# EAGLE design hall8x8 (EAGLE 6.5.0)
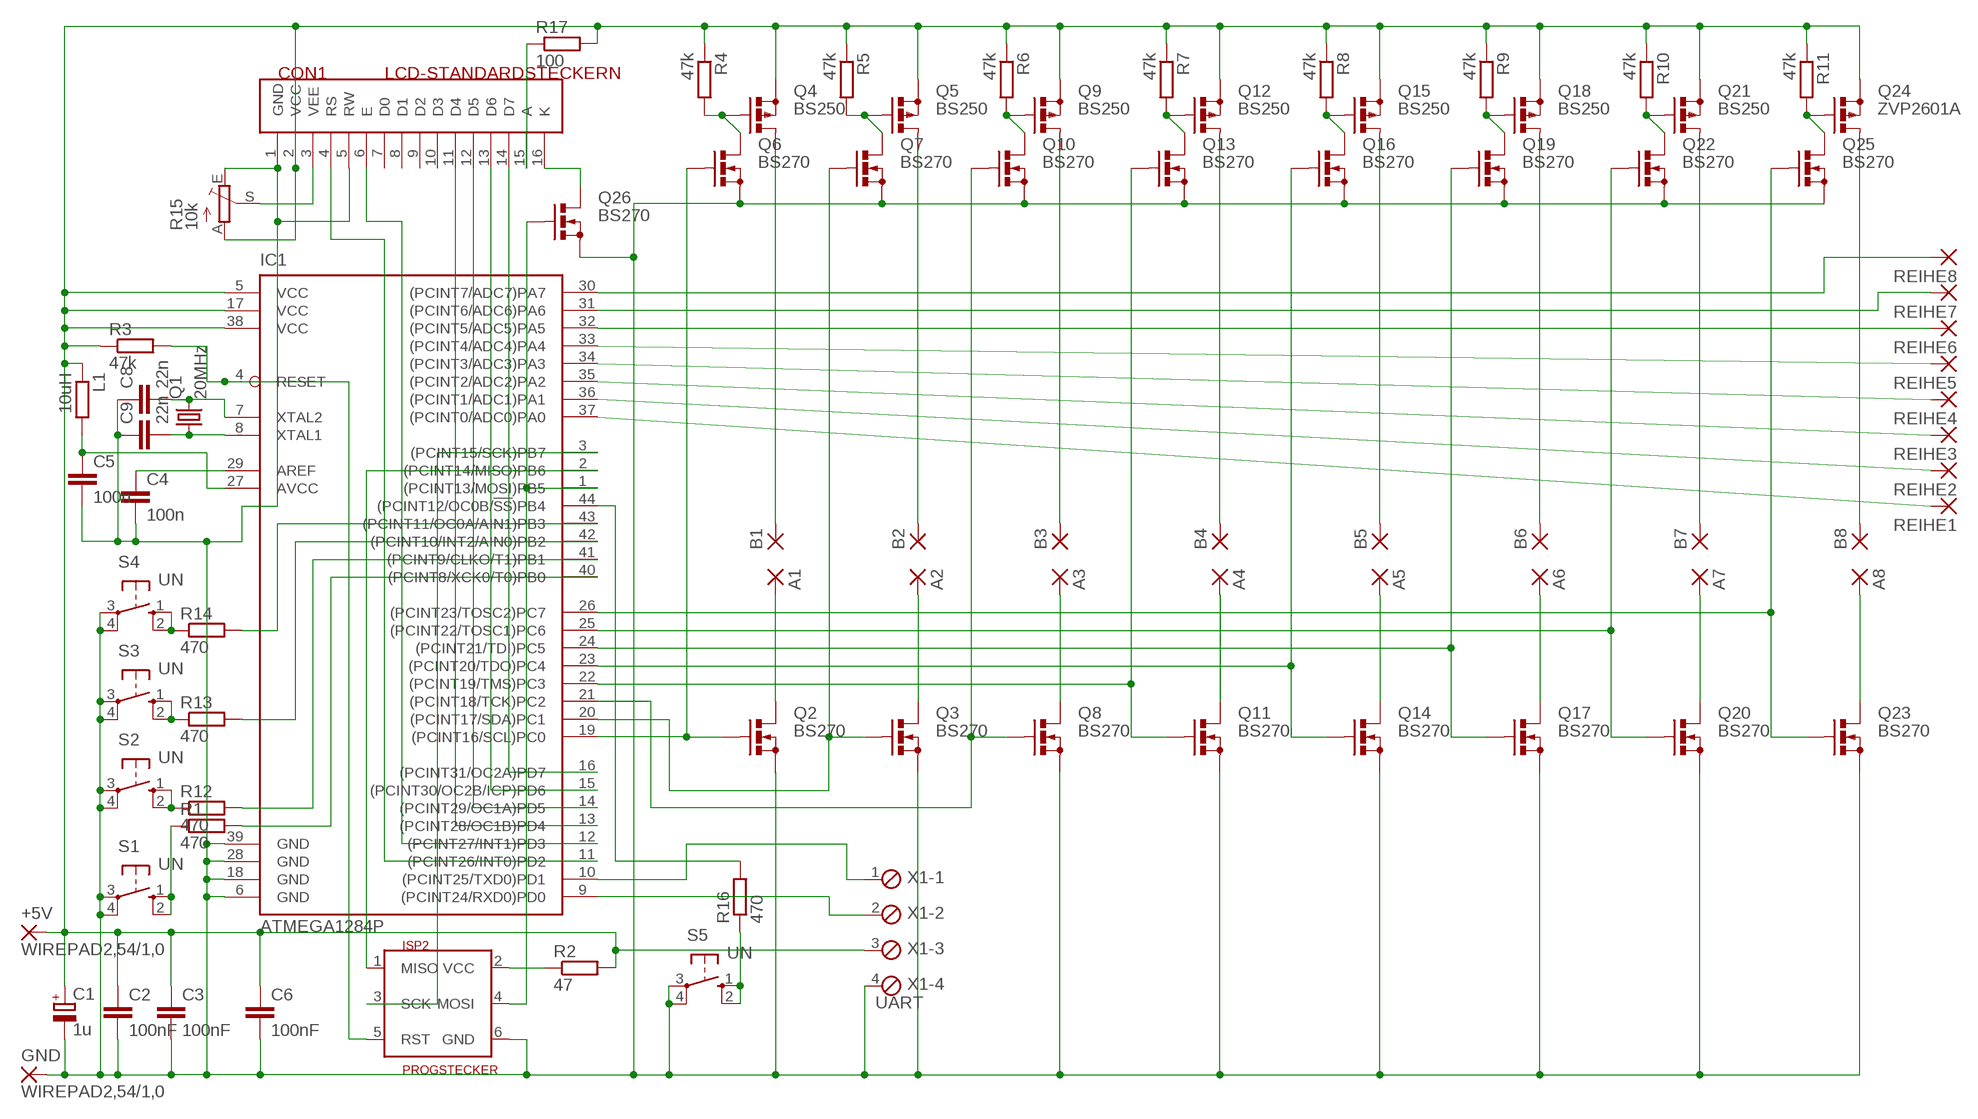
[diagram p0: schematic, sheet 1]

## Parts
+5V  WIREPAD2,54/1,0  [2,54/1,0]
A1  WIREPAD2,15/1,0  [2,15/1,0]
A2  WIREPAD2,15/1,0  [2,15/1,0]
A3  WIREPAD2,15/1,0  [2,15/1,0]
A4  WIREPAD2,15/1,0  [2,15/1,0]
A5  WIREPAD2,15/1,0  [2,15/1,0]
A6  WIREPAD2,15/1,0  [2,15/1,0]
A7  WIREPAD2,15/1,0  [2,15/1,0]
A8  WIREPAD2,15/1,0  [2,15/1,0]
B1  WIREPAD2,15/1,0  [2,15/1,0]
B2  WIREPAD2,15/1,0  [2,15/1,0]
B3  WIREPAD2,15/1,0  [2,15/1,0]
B4  WIREPAD2,15/1,0  [2,15/1,0]
B5  WIREPAD2,15/1,0  [2,15/1,0]
B6  WIREPAD2,15/1,0  [2,15/1,0]
B7  WIREPAD2,15/1,0  [2,15/1,0]
B8  WIREPAD2,15/1,0  [2,15/1,0]
C1  1u  CPOL-EUE5-6  [E5-6]
C2  100nF  C-EU025-025X050  [C025-025X050]
C3  100nF  C-EU025-025X050  [C025-025X050]
C4  100n  C-EUC1206  [C1206]
C5  100n  C-EUC1206  [C1206]
C6  100nF  C-EU025-025X050  [C025-025X050]
C8  22n  C-EUC1206  [C1206]
C9  22n  C-EUC1206  [C1206]
CON1  LCD-STANDARDSTECKERN  [STECKER16]
GND  WIREPAD2,54/1,0  [2,54/1,0]
IC1  ATMEGA1284P  ATMEGA644A  [TQFP44]
ISP2  PROGSTECKER  ISP6N  [ISP6]
L1  10uH  R-EU_0204/7  [0204/7]
Q1  20MHz  CRYSTALHC49S  [HC49/S]
Q2  BS270  BS170  [SOT54E]
Q3  BS270  BS170  [SOT54E]
Q4  BS250  [SOT54E]
Q5  BS250  [SOT54E]
Q6  BS270  BS170  [SOT54E]
Q7  BS270  BS170  [SOT54E]
Q8  BS270  BS170  [SOT54E]
Q9  BS250  [SOT54E]
Q10  BS270  BS170  [SOT54E]
Q11  BS270  BS170  [SOT54E]
Q12  BS250  [SOT54E]
Q13  BS270  BS170  [SOT54E]
Q14  BS270  BS170  [SOT54E]
Q15  BS250  [SOT54E]
Q16  BS270  BS170  [SOT54E]
Q17  BS270  BS170  [SOT54E]
Q18  BS250  [SOT54E]
Q19  BS270  BS170  [SOT54E]
Q20  BS270  BS170  [SOT54E]
Q21  BS250  [SOT54E]
Q22  BS270  BS170  [SOT54E]
Q23  BS270  BS170  [SOT54E]
Q24  ZVP2601A  BS250  [SOT54E]
Q25  BS270  BS170  [SOT54E]
Q26  BS270  BS170  [SOT54E]
R1  470  R-EU_M1406  [M1406]
R2  47  R-EU_M1406  [M1406]
R3  47k  R-EU_M1406  [M1406]
R4  47k  R-EU_M1406  [M1406]
R5  47k  R-EU_M1406  [M1406]
R6  47k  R-EU_M1406  [M1406]
R7  47k  R-EU_M1406  [M1406]
R8  47k  R-EU_M1406  [M1406]
R9  47k  R-EU_M1406  [M1406]
R10  47k  R-EU_M1406  [M1406]
R11  47k  R-EU_M1406  [M1406]
R12  470  R-EU_M1406  [M1406]
R13  470  R-EU_M1406  [M1406]
R14  470  R-EU_M1406  [M1406]
R15  10k  TRIM_EU-CA6V  [CA6V]
R16  470  R-EU_M1406  [M1406]
R17  100  R-EU_0204/7  [0204/7]
REIHE1  WIREPAD2,15/1,0  [2,15/1,0]
REIHE2  WIREPAD2,15/1,0  [2,15/1,0]
REIHE3  WIREPAD2,15/1,0  [2,15/1,0]
REIHE4  WIREPAD2,15/1,0  [2,15/1,0]
REIHE5  WIREPAD2,15/1,0  [2,15/1,0]
REIHE6  WIREPAD2,15/1,0  [2,15/1,0]
REIHE7  WIREPAD2,15/1,0  [2,15/1,0]
REIHE8  WIREPAD2,15/1,0  [2,15/1,0]
S1  UN  10-XX  [B3F-10XX]
S2  UN  10-XX  [B3F-10XX]
S3  UN  10-XX  [B3F-10XX]
S4  UN  10-XX  [B3F-10XX]
S5  UN  10-XX  [B3F-10XX]
X1  UART  MPT4  [4POL254]

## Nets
AVCC [dick]: C5.1 IC1.27(AVCC) L1.2
GND [dick]: C1.- C2.2 C3.2 C4.2 C5.2 C6.2 C8.1 C9.1 CON1.1(GND) CON1.5(RW) GND.1(P) IC1.6(GND) IC1.18(GND) IC1.28(GND) IC1.39(GND) ISP2.6(GND) Q2.S Q3.S Q6.S Q7.S Q8.S Q10.S Q11.S Q13.S Q14.S Q16.S Q17.S Q19.S Q20.S Q22.S Q23.S Q25.S Q26.S R15.E S1.3(P) S1.4(P1) S2.3(P) S2.4(P1) S3.3(P) S3.4(P1) S4.3(P) S4.4(P1) S5.3(P) S5.4(P1) X1.4
N$1: C8.2 IC1.7(XTAL2) Q1.2
N$2 [dick]: ISP2.2(VCC) R2.1
N$3 [sehrdick]: B1.1(P) Q4.D
N$4 [dick]: R1.1 S1.1(S) S1.2(S1)
N$5: C9.2 IC1.8(XTAL1) Q1.1
N$6: IC1.4(RESET) ISP2.5(RST) R3.2
N$7 [sehrdick]: B3.1(P) Q9.D
N$8: IC1.40((PCINT8/XCK0/T0)PB0) R1.2
N$9: IC1.30((PCINT7/ADC7)PA7) REIHE8.1(P)
N$10 [dick]: C4.1 IC1.29(AREF)
N$11: IC1.2((PCINT14/MISO)PB6) ISP2.1(MISO)
N$12: IC1.1((PCINT13/MOSI)PB5) ISP2.4(MOSI) Q26.G
N$13 [dick]: R12.1 S2.1(S) S2.2(S1)
N$14: IC1.3((PCINT15/SCK)PB7) ISP2.3(SCK)
N$15 [sehrdick]: B2.1(P) Q5.D
N$16: IC1.21((PCINT18/TCK)PC2) Q8.G Q10.G
N$17: IC1.31((PCINT6/ADC6)PA6) REIHE7.1(P)
N$18: Q9.G Q10.D R6.2
N$19 [sehrdick]: A1.1(P) Q2.D
N$20 [sehrdick]: A2.1(P) Q3.D
N$21: IC1.19((PCINT16/SCL)PC0) Q2.G Q6.G
N$22: IC1.20((PCINT17/SDA)PC1) Q3.G Q7.G
N$23: Q5.G Q7.D R5.2
N$24: Q4.G Q6.D R4.2
N$25 [sehrdick]: A3.1(P) Q8.D
N$26 [sehrdick]: B4.1(P) Q12.D
N$27: IC1.22((PCINT19/TMS)PC3) Q11.G Q13.G
N$28: Q12.G Q13.D R7.2
N$29 [sehrdick]: A4.1(P) Q11.D
N$30 [sehrdick]: B5.1(P) Q15.D
N$31: IC1.23((PCINT20/TDO)PC4) Q14.G Q16.G
N$32: Q15.G Q16.D R8.2
N$33 [sehrdick]: A5.1(P) Q14.D
N$34 [sehrdick]: B6.1(P) Q18.D
N$35: IC1.24((PCINT21/TDI)PC5) Q17.G Q19.G
N$36: Q18.G Q19.D R9.2
N$37 [sehrdick]: A6.1(P) Q17.D
N$38 [sehrdick]: B7.1(P) Q21.D
N$39: IC1.25((PCINT22/TOSC1)PC6) Q20.G Q22.G
N$40: Q21.G Q22.D R10.2
N$41 [sehrdick]: A7.1(P) Q20.D
N$42 [sehrdick]: B8.1(P) Q24.D
N$43: IC1.26((PCINT23/TOSC2)PC7) Q23.G Q25.G
N$44: Q24.G Q25.D R11.2
N$45 [sehrdick]: A8.1(P) Q23.D
N$46: IC1.37((PCINT0/ADC0)PA0) REIHE1.1(P)
N$47: IC1.36((PCINT1/ADC1)PA1) REIHE2.1(P)
N$48: IC1.35((PCINT2/ADC2)PA2) REIHE3.1(P)
N$49: IC1.32((PCINT5/ADC5)PA5) REIHE6.1(P)
N$50: IC1.33((PCINT4/ADC4)PA4) REIHE5.1(P)
N$51: IC1.34((PCINT3/ADC3)PA3) REIHE4.1(P)
N$52 [dick]: R13.1 S3.1(S) S3.2(S1)
N$53 [dick]: R14.1 S4.1(S) S4.2(S1)
N$54: IC1.41((PCINT9/CLKO/T1)PB1) R12.2
N$55: IC1.42((PCINT10/INT2/AIN0)PB2) R13.2
N$56: IC1.43((PCINT11/OC0A/AIN1)PB3) R14.2
N$57: CON1.3(VEE) R15.S
N$58: CON1.4(RS) IC1.11((PCINT26/INT0)PD2)
N$59: CON1.6(E) IC1.12((PCINT27/INT1)PD3)
N$60: CON1.11(D4) IC1.13((PCINT28/OC1B)PD4)
N$61: CON1.12(D5) IC1.14((PCINT29/OC1A)PD5)
N$62: CON1.13(D6) IC1.15((PCINT30/OC2B/ICP)PD6)
N$63: CON1.14(D7) IC1.16((PCINT31/OC2A)PD7)
N$64 [sehrdick]: CON1.16(K) Q26.D
N$65 [dick]: R16.1 S5.1(S) S5.2(S1)
N$66: IC1.44((PCINT12/OC0B/!SS!)PB4) R16.2
N$67 [sehrdick]: CON1.15(A) R17.1
N$68: IC1.9((PCINT24/RXD0)PD0) X1.2
N$69: IC1.10((PCINT25/TXD0)PD1) X1.1
VCC [dick]: +5V.1(P) C1.+ C2.1 C3.1 C6.1 CON1.2(VCC) IC1.5(VCC) IC1.17(VCC) IC1.38(VCC) L1.1 Q4.S Q5.S Q9.S Q12.S Q15.S Q18.S Q21.S Q24.S R2.2 R3.1 R4.1 R5.1 R6.1 R7.1 R8.1 R9.1 R10.1 R11.1 R15.A R17.2 X1.3
Unconnected: CON1.7(D0) CON1.8(D1) CON1.9(D2) CON1.10(D3)

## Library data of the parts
+5V A1-A8 B1-B8 GND REIHE1-REIHE8 = wirepad:WIREPAD: Wire PAD connect wire on PCB
C1 = resistor:CPOL-EU: POLARIZED CAPACITOR, European symbol
C2-C6 C8 C9 = rcl:C-EU: CAPACITOR, European symbol
CON1 = 6_stecker:LCD-STANDARDSTECKER: Standard-Stecker fuer die meisten LCD-Module
IC1 = atmel:ATMEGA644: 8-bit Microcontroller with 64K Bytes In-System Programmable Flash Source: http://www.atmel.com/dyn/resources/prod_documents/doc2593.pdf; MPN: ATMEGA644PV-10AU; OC_FARNELL: 1455123; OC_NEWARK: 58M3748
ISP2 = stecker:ISP6: ISP-Stecker 6polig
L1 R1-R14 R16 R17 = rcl:R-EU_: RESISTOR, European symbol
Q1 = crystal:CRYSTAL: CRYSTAL
Q2 Q3 Q6-Q8 Q10 Q11 Q13 Q14 Q16 Q17 Q19 Q20 Q22 Q23 Q25 Q26 = transistor-small-signal:BS170: N-CHANNEL MOS FET
Q4 Q5 Q9 Q12 Q15 Q18 Q21 Q24 = transistor-small-signal:BS250: P-CHANNEL MOS FET
R15 = pot:TRIM_EU-: POTENTIOMETER
S1-S5 = switch-omron:10-XX: OMRON SWITCH; MPN: B3F-1000; OC_FARNELL: 176432; OC_NEWARK: 36M3542
X1 = con-phoenix-254:MPT4: PHOENIX CONNECTOR; OC_FARNELL: unknown; OC_NEWARK: unknown

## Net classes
1 dick: width 0.508 mm
2 sehrdick: width 1.016 mm

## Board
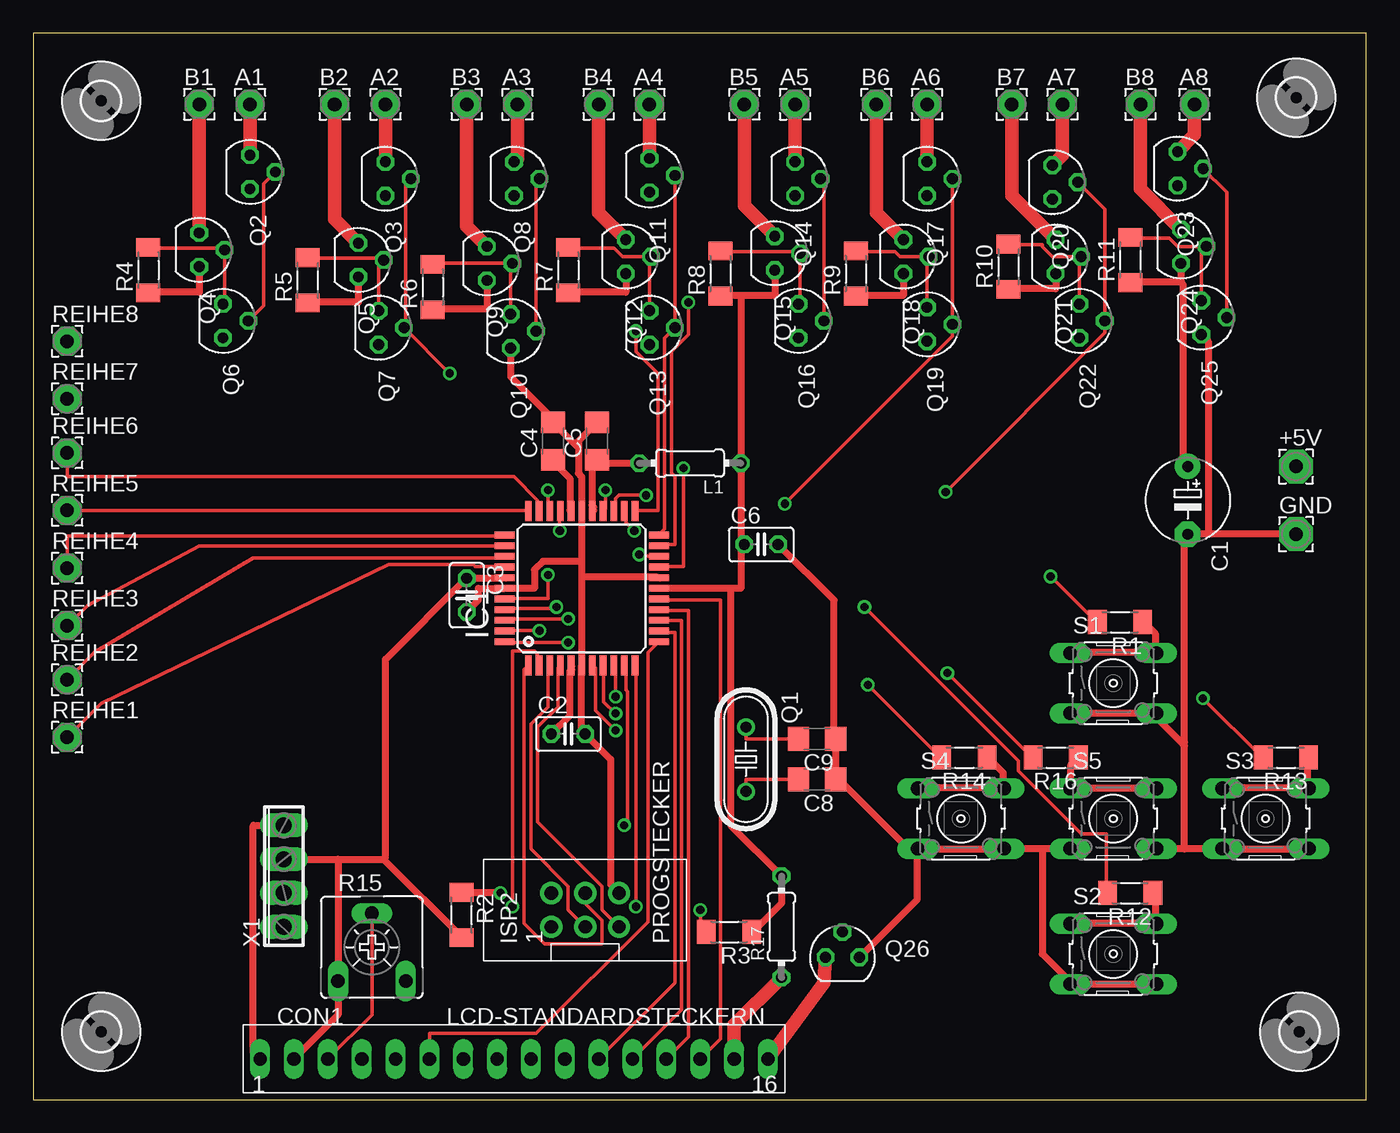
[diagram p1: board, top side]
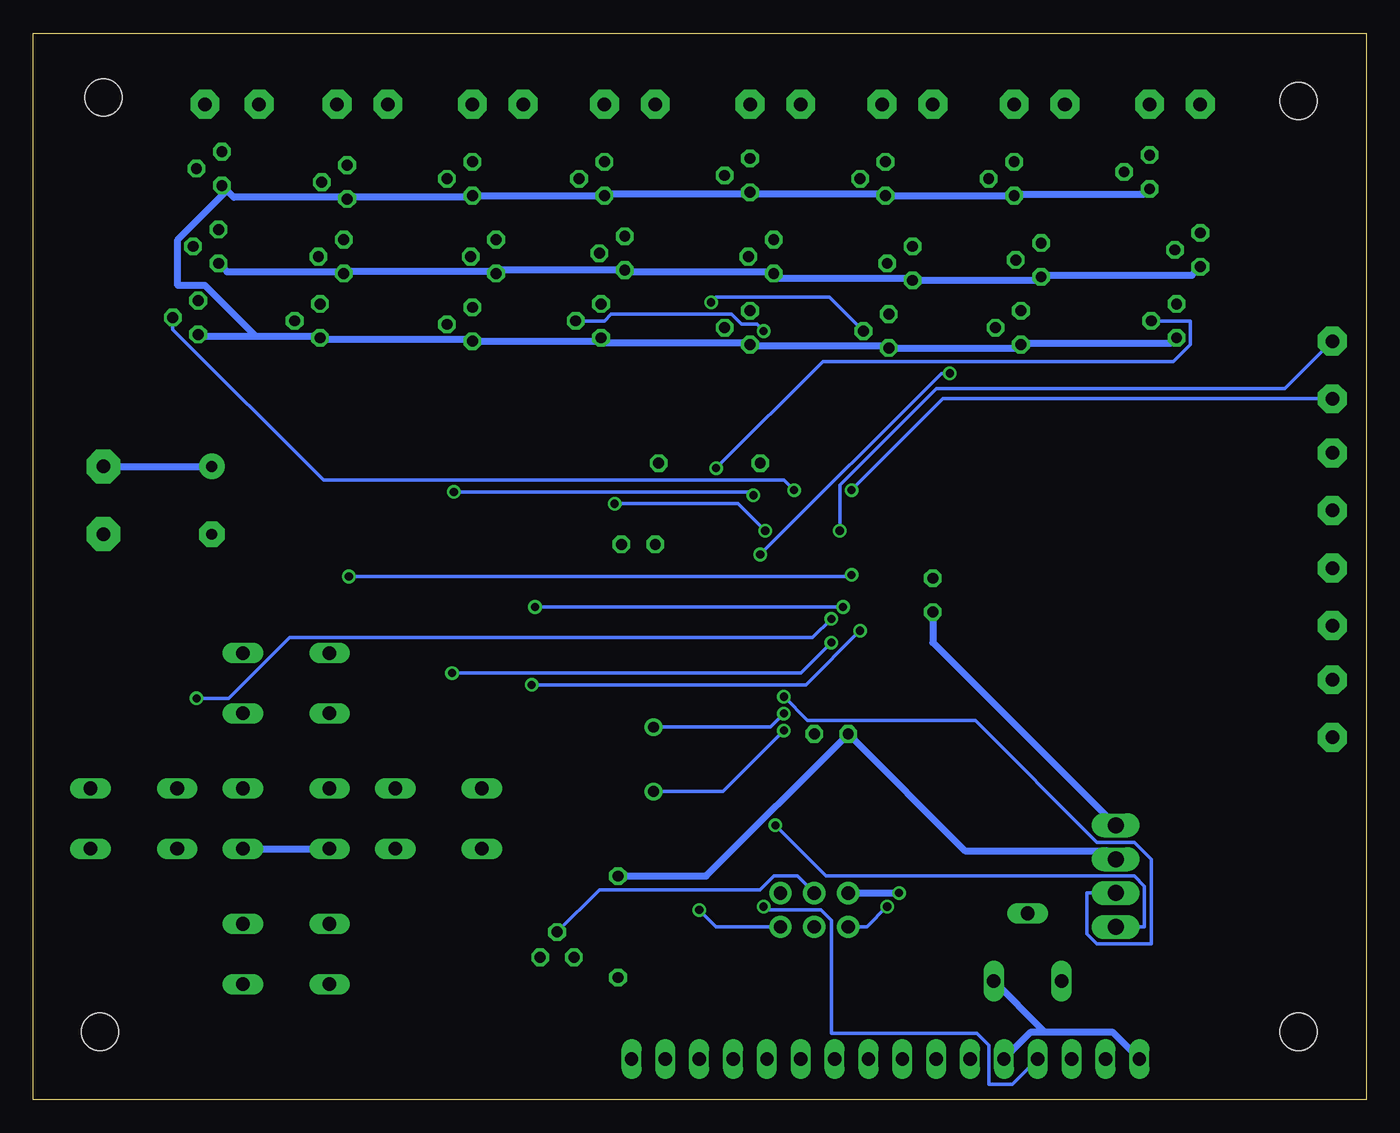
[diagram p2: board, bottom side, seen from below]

Size 100 x 80 mm. Coordinates in mm from the lower left corner, seen from the top.
Outline: 0,0 100,0 100,80 0,80 0,0
Copper layers (1*16): Top 0.035mm / dielectric 1.5mm / Bottom 0.035mm
Design rules "default": minimum track width 10mil, minimum drill 24mil, track to track 8mil, track to pad 8mil, pad to pad 8mil, via to via 8mil, smd to smd 8mil, copper to edge 40mil, drill to drill 8mil, minimum pad ring 10mil, minimum via ring 8mil, stop-mask expansion 4mil, vias tented up to drill 0mil, thermal gap 10mil

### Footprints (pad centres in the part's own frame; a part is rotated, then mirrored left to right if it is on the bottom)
2,54/1,0 = drill 1.016 pad 2.54 octagon: 1 0,0
2,15/1,0 = drill 1.016 pad 2.159 octagon: 1 0,0
E5-6 = drill 0.813 pad 1.905: + -2.54,0 | drill 0.813 pad 1.905 octagon: - 2.54,0
C025-025X050 = drill 0.813 octagon: 1 -1.27,0; 2 1.27,0
C1206 = smd 1.6 x 1.8: 1 -1.4,0; 2 1.4,0
STECKER16 = drill 1 long: 1 -17.78,0; 2 -15.24,0; 3 -12.7,0; 4 -10.16,0; 5 -7.62,0; 6 -5.08,0; 7 -2.54,0; 8 0,0; 9 2.54,0; 10 5.08,0; 11 7.62,0; 12 10.16,0; 13 12.7,0; 14 15.24,0; 15 17.78,0; 16 20.32,0
TQFP44 = smd 1.5 x 0.5: 1 -5.8,4; 2 -5.8,3.2; 3 -5.8,2.4; 4 -5.8,1.6; 5 -5.8,0.8; 6 -5.8,0; 7 -5.8,-0.8; 8 -5.8,-1.6; 9 -5.8,-2.4; 10 -5.8,-3.2; 11 -5.8,-4; 23 5.8,-4; 24 5.8,-3.2; 25 5.8,-2.4; 26 5.8,-1.6; 27 5.8,-0.8; 28 5.8,0; 29 5.8,0.8; 30 5.8,1.6; 31 5.8,2.4; 32 5.8,3.2; 33 5.8,4 | smd 0.5 x 1.5: 12 -4,-5.8; 13 -3.2,-5.8; 14 -2.4,-5.8; 15 -1.6,-5.8; 16 -0.8,-5.8; 17 0,-5.8; 18 0.8,-5.8; 19 1.6,-5.8; 20 2.4,-5.8; 21 3.2,-5.8; 22 4,-5.8; 34 4,5.8; 35 3.2,5.8; 36 2.4,5.8; 37 1.6,5.8; 38 0.8,5.8; 39 0,5.8; 40 -0.8,5.8; 41 -1.6,5.8; 42 -2.4,5.8; 43 -3.2,5.8; 44 -4,5.8
ISP6 = drill 1 pad 1.676: 1 -1.27,2.54; 2 1.27,2.54; 3 -1.27,0; 4 1.27,0; 5 -1.27,-2.54; 6 1.27,-2.54
0204/7 = drill 0.813 octagon: 1 -3.81,0; 2 3.81,0
HC49/S = drill 0.813: 1 -2.413,0; 2 2.413,0
SOT54E = drill 0.813 octagon: D -1.27,0; G 0,1.905; S 1.27,0
M1406 = smd 1.4 x 1.8: 1 -1.7,0; 2 1.7,0
CA6V = drill 1.016 long: A -2.54,-2.54; E 2.54,-2.54; S 0,2.54
B3F-10XX = drill 1.016 long: 1 -3.251,2.261; 2 3.251,2.261; 3 -3.251,-2.261; 4 3.251,-2.261
2,8 = hole 2.8: 0,0
4POL254 = drill 1.2 long: 1 -3.81,0; 2 -1.27,0; 3 1.27,0; 4 3.81,0

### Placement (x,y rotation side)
+5V  94.74,47.5 0 top
A1  16.26,74.68 0 top
A2  26.42,74.68 0 top
A3  36.32,74.68 0 top
A4  46.23,74.68 0 top
A5  57.15,74.68 0 top
A6  67.06,74.68 0 top
A7  77.22,74.68 0 top
A8  87.12,74.68 0 top
B1  12.45,74.68 0 top
B2  22.61,74.68 0 top
B3  32.51,74.68 0 top
B4  42.42,74.68 0 top
B5  53.34,74.68 0 top
B6  63.25,74.68 0 top
B7  73.41,74.68 0 top
B8  83.06,74.68 0 top
C1  86.61,44.96 270 top
C2  40.13,27.43 0 top
C3  32.51,37.85 270 top
C4  38.99,49.4 90 top
C5  42.29,49.4 90 top
C6  54.61,41.66 0 top
C8  58.8,24 180 top
C9  58.8,27.05 180 top
CON1  34.8,3.05 0 top
GND  94.74,42.42 0 top
IC1  41.15,38.35 90 top
ISP2  41.4,14.22 90 top
L1  49.28,47.75 180 top
Q1  53.47,25.53 270 top
Q2  16.26,69.6 270 top
Q3  26.42,69.09 270 top
Q4  12.45,63.75 270 top
Q5  24.38,62.99 270 top
Q6  14.22,58.42 270 top
Q7  25.91,57.91 270 top
Q8  36.07,69.09 270 top
Q9  34.04,62.74 270 top
Q10  35.81,57.66 270 top
Q11  46.23,69.34 270 top
Q12  44.45,63.25 270 top
Q13  46.23,57.91 270 top
Q14  57.15,69.09 270 top
Q15  55.63,63.5 270 top
Q16  57.4,58.42 270 top
Q17  67.06,69.09 270 top
Q18  65.28,63.25 270 top
Q19  67.06,58.17 270 top
Q20  76.45,68.83 270 top
Q21  76.71,63.25 270 top
Q22  78.49,58.42 270 top
Q23  85.85,69.85 270 top
Q24  86.11,64.01 270 top
Q25  87.63,58.67 270 top
Q26  60.71,10.67 0 top
R1  81.53,35.81 180 top
R2  32.13,13.84 270 top
R3  52.2,12.57 180 top
R4  8.64,62.23 90 top
R5  20.57,61.47 90 top
R6  29.97,60.96 90 top
R7  40.13,62.23 90 top
R8  51.56,61.98 90 top
R9  61.72,61.98 90 top
R10  73.15,62.48 90 top
R11  82.3,62.99 90 top
R12  82.3,15.49 180 top
R13  93.98,25.65 180 top
R14  69.85,25.65 180 top
R15  25.4,11.43 0 top
R16  76.71,25.65 180 top
R17  56.13,12.95 90 top
REIHE1  2.54,27.18 0 top
REIHE2  2.54,31.5 0 top
REIHE3  2.54,35.56 0 top
REIHE4  2.54,39.88 0 top
REIHE5  2.54,44.2 0 top
REIHE6  2.54,48.51 0 top
REIHE7  2.54,52.58 0 top
REIHE8  2.54,56.9 0 top
S1  81.03,31.24 0 top
S2  81.03,10.92 0 top
S3  92.46,21.08 0 top
S4  69.6,21.08 0 top
S5  81.03,21.08 0 top
U$1  [2,8]  95,5.08 0 top
U$2  [2,8]  5.08,5.08 0 top
U$3  [2,8]  5.08,74.93 0 top
U$4  [2,8]  94.74,75.18 0 top
X1  18.8,16.76 90 top

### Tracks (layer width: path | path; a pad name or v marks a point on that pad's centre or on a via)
AVCC
  Top 0.508: 42.04,44.2 IC1.27 42.04,44.45 41.91,44.58 41.91,47.5 42.29,47.88 C5.1 42.42,47.75 L1.2
GND
  Top 0.508: X1.4 16.51,20.57 16.51,3.56 CON1.1 | 41.15,32.51 IC1.6 | IC1.6 41.15,27.69 C2.2 43.31,25.53 43.31,16.13 ISP2.6 | 35.43,38.35 IC1.39 | IC1.39 33.4,38.35 33.4,37.47 C3.2 | 46.99,39.12 IC1.18 46.74,39.24 41.15,39.24 | 41.15,44.2 IC1.28 | IC1.28 41.15,46.74 40.89,46.99 40.89,49.02 | 40.89,49.02 40.89,49.4 C5.2 | IC1.28 41.15,40.39 | 41.15,40.39 41.15,39.24 | 40.89,49.02 40.77,49.02 C4.2 38.99,51.05 35.81,54.23 Q10.S | IC1.39 37.59,38.35 37.59,39.75 38.23,40.39 41.15,40.39 | 41.15,39.24 IC1.6 | S2.4 84.2,8.64 77.85,8.64 S2.3 77.72,8.89 75.69,10.92 75.69,18.8 | 75.69,18.8 77.72,18.8 S5.3 | 75.69,18.8 72.9,18.8 S4.4 72.64,18.8 66.55,18.8 S4.3 | Q26.S 66.29,14.99 66.29,18.8 S4.3 | S4.3 66.17,18.29 60.45,24 C8.1 C9.1 60.07,27.18 60.07,37.47 C6.2 | GND.1 88.14,42.42 | 88.14,42.42 C1.- 86.36,42.16 86.36,26.8 86.23,26.67 | S1.3 77.85,28.96 84.2,28.96 S1.4 84.2,28.7 86.23,26.67 | 86.36,18.8 89.15,18.8 S3.3 89.41,18.8 95.63,18.8 S3.4 | 86.36,18.8 84.33,18.8 S5.4 | 86.23,26.67 86.36,26.54 86.36,18.8 | 88.14,42.42 88.14,56.9 Q25.S
  Bottom 0.508: CON1.1 19.05,5.08 24.26,5.08 | 24.26,5.08 25.15,5.08 CON1.5 | R15.E 24.26,5.21 24.26,5.08 | X1.4 32.51,34.29 C3.2 | S5.3 77.85,18.8 84.2,18.8 S5.4 | Q2.S 16.64,67.94 26.29,67.94 Q3.S Q8.S 36.2,67.94 46.1,67.94 Q11.S 46.35,67.94 57.02,67.94 Q14.S Q17.S 67.18,67.69 76.33,67.69 Q20.S 76.58,67.69 84.96,67.69 Q23.S 85.6,68.07 89.15,64.52 89.15,61.09 87.12,61.09 83.44,57.4 83.44,57.28 | 83.44,57.28 87.5,57.28 Q25.S | 83.44,57.28 78.61,57.28 Q22.S 78.36,57.02 67.18,57.02 Q19.S 57.66,56.9 Q16.S 57.02,56.77 46.35,56.77 Q13.S 46.1,56.52 35.94,56.52 Q10.S 26.16,56.39 Q7.S 25.78,56.77 14.61,56.77 Q6.S
N$1  (via drill 0.61)
  Top 0.254: v43.69,27.69 42.16,29.21 42.16,32.38 42.04,32.51 IC1.7 | C8.2 53.47,24 Q1.2
  Bottom 0.254: v43.69,27.69 48.26,23.11 Q1.2
N$2  (via drill 0.61)
  Top 0.508: v35.05,15.49 32.13,15.49 R2.1
  Bottom 0.508: ISP2.2 v35.05,15.49
N$3
  Top 1.016: B1.1 Q4.D
N$4
  Top 0.508: R1.1 83.31,35.81 84.2,34.92 84.2,33.53 S1.2 83.95,33.53 77.85,33.53 S1.1
N$5  (via drill 0.61)
  Top 0.254: v43.69,28.96 42.8,29.84 42.8,32.51 IC1.8 | C9.2 53.47,27.05 Q1.1
  Bottom 0.254: v43.69,28.96 44.7,27.94 Q1.1
N$6  (via drill 0.61)
  Top 0.254: ISP2.5 42.67,14.22 42.67,16 37.85,20.83 37.85,27.94 39.37,29.46 39.37,32.38 39.5,32.51 IC1.4 | v50.04,14.22 50.04,12.95 50.42,12.57 R3.2
  Bottom 0.254: v50.04,14.22 48.77,12.95 ISP2.5
N$7
  Top 1.016: Q9.D 32.51,65.53 B3.1
N$8  (via drill 0.61)
  Top 0.254: v38.61,39.37 38.61,37.59 35.43,37.59 IC1.40 | v76.33,39.24 79.76,35.81 R1.2
  Bottom 0.254: v38.61,39.37 38.73,39.24 v76.33,39.24
N$9  (via drill 0.61)
  Top 0.254: v39.5,42.67 39.5,44.07 IC1.30
  Bottom 0.254: v39.5,42.67 39.5,46.1 32.26,53.34 6.1,53.34 REIHE8.1
N$10
  Top 0.508: IC1.29 40.26,44.2 40.26,46.61 38.99,47.88 C4.1
N$11  (via drill 0.61)
  Top 0.254: v35.94,14.48 35.94,33.66 37.59,33.66 37.85,33.4 37.85,32.64 IC1.2
  Bottom 0.254: v35.94,14.48 37.47,12.95 ISP2.1
N$12
  Top 0.254: ISP2.4 41.4,14.73 42.67,13.46 42.67,11.68 38.35,11.68 36.83,13.21 36.83,32.26 37.08,32.51 IC1.1
  Bottom 0.254: Q26.G 57.53,15.75 45.47,15.75 44.45,16.76 42.67,16.76 ISP2.4
N$13
  Top 0.508: R12.1 84.07,15.49 84.2,15.37 84.2,13.21 S2.2 83.95,13.21 77.85,13.21 S2.1
N$14
  Top 0.254: ISP2.3 40.13,14.22 40.13,16 37.34,18.8 37.34,28.19 38.61,29.46 38.61,32.38 38.73,32.51 IC1.3
N$15
  Top 1.016: Q5.D 22.61,66.04 B2.1
N$16  (via drill 0.61)
  Top 0.254: v49.15,59.82 49.15,57.4 47.88,56.13 47.88,46.99 48.13,46.74 48.13,41.66 46.99,41.66 IC1.21 | Q8.G 37.72,68.83 Q10.G
  Bottom 0.254: v49.15,59.82 48.77,60.2 40.26,60.2 Q10.G
N$17  (via drill 0.61)
  Top 0.254: v38.61,45.72 38.61,44.32 38.73,44.2 IC1.31
  Bottom 0.254: v38.61,45.72 31.75,52.58 REIHE7.1
N$18
  Top 0.254: 35.81,62.74 29.97,62.74 R6.2 | 35.81,62.74 Q10.D | 35.81,62.74 Q9.G
N$19
  Top 1.016: A1.1 Q2.D
N$20
  Top 1.016: A2.1 Q3.D
N$21  (via drill 0.61)
  Top 0.254: v48.77,47.37 48.77,40.01 46.99,40.01 IC1.19 | Q2.G 17.27,68.71 17.27,59.56 Q6.G
  Bottom 0.254: v48.77,47.37 40.77,55.37 14.48,55.37 13.21,56.64 13.21,58.42 Q6.G
N$22  (via drill 0.61)
  Top 0.254: v45.47,40.89 45.47,40.77 46.86,40.77 IC1.20 | v31.24,54.48 Q7.G 27.94,57.91 27.94,68.71 Q3.G
  Bottom 0.254: v45.47,40.89 31.88,54.48 v31.24,54.48
N$23
  Top 0.254: 25.91,63.12 26.29,63.12 Q5.G 25.91,63.12 | 25.91,63.12 20.57,63.12 R5.2 | 25.91,63.12 Q7.D
N$24
  Top 0.254: R4.2 8.64,63.88 14.35,63.88 Q4.G 14.35,59.82 Q6.D
N$25
  Top 1.016: Q8.D 36.32,70.61 A3.1
N$26
  Top 1.016: Q12.D 42.42,66.55 B4.1
N$27
  Top 0.254: IC1.22 46.99,42.42 47.37,42.8 47.37,57.15 Q13.G Q11.G
N$28
  Top 0.254: 46.23,63.25 44.2,63.25 43.56,63.88 40.13,63.88 R7.2 | 46.23,63.25 Q13.D | 46.23,63.25 Q12.G
N$29
  Top 1.016: A4.1 Q11.D
N$30
  Top 1.016: Q15.D 53.34,67.06 B5.1
N$31  (via drill 0.61)
  Top 0.254: v45.21,57.66 45.21,56.13 46.86,54.48 46.86,44.2 45.21,44.2 IC1.23 | Q14.G 59.31,68.83 Q16.G
  Bottom 0.254: v45.21,57.66 45.72,58.17 46.86,58.17 47.62,58.93 56.64,58.93 57.15,58.42 Q16.G
N$32
  Top 0.254: R8.2 51.56,63.63 57.53,63.63 Q15.G 57.53,59.82 Q16.D
N$33
  Top 1.016: A5.1 Q14.D
N$34
  Top 1.016: Q18.D 63.25,66.55 B6.1
N$35  (via drill 0.61)
  Top 0.254: v45.09,42.67 44.45,43.31 44.45,44.07 IC1.24 | v56.39,44.7 68.96,57.28 Q19.G Q17.G
  Bottom 0.254: v45.09,42.67 47.12,44.7 v56.39,44.7
N$36
  Top 0.254: 67.06,63.25 65.02,63.25 64.64,63.63 61.72,63.63 R9.2 | 67.06,63.25 Q19.D | 67.06,63.25 Q18.G
N$37
  Top 1.016: A6.1 Q17.D
N$38
  Top 1.016: Q21.D 73.41,67.82 B7.1
N$39  (via drill 0.61)
  Top 0.254: v45.97,45.34 43.94,45.34 43.69,45.09 43.69,44.32 43.56,44.2 IC1.25 | v68.45,45.59 80.39,57.53 Q22.G 80.39,66.8 Q20.G
  Bottom 0.254: v45.97,45.34 46.23,45.59 v68.45,45.59
N$40
  Top 0.254: 78.49,63.25 76.45,63.25 75.69,64.01 75.69,64.14 73.15,64.14 R10.2 | 78.49,63.25 Q22.D | 78.49,63.25 Q21.G
N$41
  Top 1.016: Q20.D 77.22,70.87 A7.1
N$42
  Top 1.016: Q24.D 83.06,68.33 B8.1
N$43  (via drill 0.61)
  Top 0.254: v42.93,45.72 42.93,44.32 42.8,44.2 IC1.26 | Q23.G 89.53,68.07 Q25.G
  Bottom 0.254: v42.93,45.72 43.69,46.48 78.23,46.48 89.53,57.78 Q25.G
N$44
  Top 0.254: 87.63,64.01 85.85,64.01 85.22,64.64 82.3,64.64 R11.2 | 87.63,64.01 Q25.D | 87.63,64.01 Q24.G
N$45
  Top 1.016: Q23.D 87.12,72.39 A8.1
N$46
  Top 0.254: REIHE1.1 5.08,29.72 26.67,40.13 33.02,40.13 33.15,40.01 35.31,40.01 IC1.37
N$47
  Top 0.254: REIHE2.1 4.57,33.53 16.51,40.64 35.31,40.64 IC1.36
N$48
  Top 0.254: REIHE3.1 4.06,37.08 12.45,41.53 35.31,41.53 IC1.35
N$49
  Top 0.254: REIHE6.1 2.54,46.74 36.07,46.74 37.85,44.96 37.85,44.2 IC1.32
N$50
  Top 0.254: REIHE5.1 37.08,44.2 IC1.33
N$51
  Top 0.254: REIHE4.1 2.54,42.29 35.31,42.29 IC1.34
N$52
  Top 0.508: R13.1 95.63,25.65 95.63,23.37 S3.2 95.38,23.37 89.28,23.37 S3.1
N$53
  Top 0.508: R14.1 71.63,25.65 72.77,24.51 72.77,23.37 S4.2 72.52,23.37 66.42,23.37 S4.1
N$54  (via drill 0.61)
  Top 0.254: v39.24,36.96 39.24,36.83 35.43,36.83 IC1.41 | v62.36,36.96 73.91,25.4 73.91,24.64 78.61,19.94 80.52,19.94 80.52,15.49 R12.2
  Bottom 0.254: v62.36,36.96 v39.24,36.96
N$55  (via drill 0.61)
  Top 0.254: v40.13,36.07 35.43,36.07 IC1.42 | v87.76,30.1 92.2,25.65 R13.2
  Bottom 0.254: v40.13,36.07 41.53,34.67 80.77,34.67 85.34,30.1 v87.76,30.1
N$56  (via drill 0.61)
  Top 0.254: v37.97,35.18 35.43,35.18 IC1.43 | v62.61,31.11 68.07,25.65 R14.2
  Bottom 0.254: v37.97,35.18 42.04,31.11 v62.61,31.11
N$57
  Top 0.254: CON1.3 25.4,6.35 R15.S
N$58  (via drill 0.61)
  Top 0.254: v45.21,14.48 45.21,32.51 IC1.11
  Bottom 0.254: v45.21,14.48 44.96,14.22 40.89,14.22 40.13,13.46 40.13,4.95 29.21,4.95 28.32,4.06 28.32,1.14 26.54,1.14 CON1.4
N$59
  Top 0.254: CON1.6 29.72,4.95 37.72,4.95 46.1,13.34 46.1,33.53 46.86,34.29 IC1.12
N$60
  Top 0.254: CON1.11 48.13,8.76 48.13,35.05 46.99,35.05 IC1.13
N$61
  Top 0.254: CON1.12 48.64,6.73 48.64,35.94 46.99,35.94 IC1.14
N$62
  Top 0.254: CON1.13 49.15,4.7 49.15,36.7 46.99,36.7 IC1.15
N$63
  Top 0.254: CON1.14 51.56,4.57 51.56,37.47 46.99,37.47 IC1.16
N$64
  Top 1.016: Q26.D 59.31,8.76 CON1.16
N$65
  Top 0.508: R16.1 78.36,25.65 77.85,25.15 77.85,23.37 S5.1 78.11,23.37 84.2,23.37 S5.2
N$66  (via drill 0.61)
  Top 0.254: v40.13,34.29 35.43,34.29 IC1.44 | v68.58,32 74.93,25.65 R16.2
  Bottom 0.254: v40.13,34.29 42.42,32 v68.58,32
N$67
  Top 1.016: R17.1 52.58,5.59 CON1.15
N$68  (via drill 0.61)
  Top 0.254: v43.69,30.23 43.69,32.38 43.56,32.51 IC1.9
  Bottom 0.254: v43.69,30.23 41.91,28.45 29.34,28.45 20.19,19.3 17.4,19.3 16.13,18.03 16.13,11.68 20.19,11.68 20.95,12.45 20.95,15.49 X1.2
N$69  (via drill 0.61)
  Top 0.254: v44.32,20.57 44.58,20.83 44.58,30.61 44.45,30.73 44.45,32.51 IC1.10
  Bottom 0.254: v44.32,20.57 40.51,16.76 17.4,16.76 16.64,16 16.64,12.95 X1.1
VCC
  Top 0.508: CON1.2 22.86,6.35 R15.A 22.86,18.03 | 35.43,39.12 IC1.38 35.18,39.12 C3.1 26.42,33.02 26.42,18.16 26.29,18.03 | 26.29,18.03 32.13,12.19 R2.2 | X1.3 22.86,18.03 | 22.86,18.03 26.29,18.03 | Q12.S 44.45,60.58 40.13,60.58 R7.1 | Q4.S 12.45,60.58 8.64,60.58 R4.1 | Q5.S 24.38,59.82 20.57,59.82 R5.1 | Q9.S 34.04,59.31 29.97,59.31 R6.1 | 40.39,32.51 IC1.5 40.39,32.26 40.26,32.13 40.26,28.83 C2.1 | R3.1 53.98,12.57 56.13,14.73 R17.2 52.32,20.57 52.32,38.35 | 46.99,38.35 IC1.17 52.32,38.35 | 52.32,38.35 53.09,38.35 53.09,41.66 | 53.09,41.66 L1.1 53.09,60.33 | Q21.S 76.71,60.83 73.15,60.83 R10.1 | 86.11,61.34 82.3,61.34 R11.1 | Q24.S 86.11,61.34 | Q18.S 65.28,60.33 61.72,60.33 R9.1 | 53.09,60.33 55.63,60.33 Q15.S | 53.09,60.33 51.56,60.33 R8.1 | C1.+ 86.23,47.88 86.23,61.21 86.11,61.34 | C6.1 53.09,41.66
  Bottom 0.508: Q4.S 13.08,61.85 24.26,61.85 Q5.S 24.64,61.47 Q9.S 34.16,61.59 44.07,61.59 Q12.S 44.58,62.1 55.5,62.1 Q15.S 65.02,62.23 Q18.S 65.41,62.1 76.58,62.1 Q21.S 76.83,62.1 85.47,62.1 Q24.S | R17.2 49.53,16.76 C2.1 30.1,18.67 19.43,18.67 X1.3 | +5V.1 C1.+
